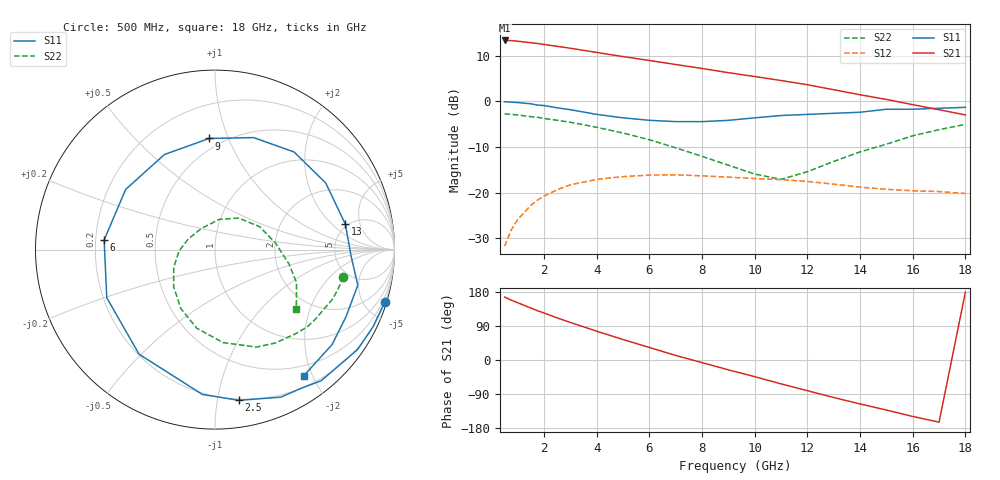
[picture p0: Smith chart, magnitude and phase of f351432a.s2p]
!ATF-35143
!S-PARAMETERS at Vds=2V  Id=5mA.  LAST UPDATED 06-3-99
# ghz s ma r 50
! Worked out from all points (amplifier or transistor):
!   23 points, 500 MHz to 18 GHz, reference 50 ohm
!   highest |S21| = 13.3 dB at 500 MHz (marker M1)
!   |S21| within 3 dB of that: start of sweep to 4.414 GHz
!   unconditionally stable (mu >= 1): 9.019 GHz to end of sweep
!   at 1.5 GHz: K = 0.17, MSG = 17.8 dB, |S12| = -22.7 dB
!   at 7 GHz: K = 0.78, MSG = 12.1 dB, |S12| = -16.1 dB
!   at 18 GHz: K = 1.55, MAG = 4.2 dB, |S12| = -20.2 dB
!   lowest NFmin = 0.10 dB at 500 MHz
!   S11 on the Smith chart (normalised r, x): 500 MHz: 0.23, -6.68; 2.5 GHz: 0.19, -1.15; 6 GHz: 0.23, +0.04; 9 GHz: 0.42, +0.85; 13 GHz: 4.77, +2.98; 18 GHz: 0.35, -1.87
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0.5  0.99 -17.0  4.64 166.0  0.026 78.0  0.73 -12.0
0.75  0.98 -26.0  4.62 158.0  0.039 71.0  0.72 -18.0
1  0.97 -35.0  4.55 151.0  0.051 66.0  0.71 -23.0
1.5  0.94 -51.0  4.38 137.0  0.073 55.0  0.68 -35.0
1.75  0.91 -58.0  4.3 130.0  0.083 50.0  0.67 -40.0
2.5  0.85 -81.0  4 111.0  0.108 35.0  0.62 -57.0
3  0.81 -95.0  3.81 99.0  0.122 25.0  0.59 -67.0
4  0.72 -126.0  3.43 76.0  0.14 7.0  0.52 -85.0
5  0.66 -156.0  3.09 54.0  0.15 -10.0  0.45 -103.0
6  0.62 175.0  2.8 33.0  0.156 -26.0  0.38 -120.0
7  0.6 146.0  2.53 12.0  0.157 -41.0  0.31 -138.0
8  0.6 118.0  2.29 -7.0  0.153 -54.0  0.25 -157.0
9  0.62 93.0  2.06 -26.0  0.148 -67.0  0.2 -178.0
10  0.66 71.0  1.87 -44.0  0.143 -78.0  0.16 158.0
11  0.7 51.0  1.69 -63.0  0.139 -89.0  0.14 122.0
12  0.72 31.0  1.52 -81.0  0.133 -100.0  0.17 82.0
13  0.74 11.0  1.34 -99.0  0.124 -111.0  0.22 53.0
14  0.76 -3.0  1.18 -116.0  0.115 -119.0  0.28 27.0
15  0.82 -14.0  1.05 -132.0  0.109 -127.0  0.34 6.0
16  0.82 -27.0  0.92 -149.0  0.105 -135.0  0.42 -11.0
17  0.84 -39.0  0.81 -164.0  0.103 -143.0  0.49 -22.0
18  0.86 -55.0  0.71 179.0  0.098 -152.0  0.56 -36.0
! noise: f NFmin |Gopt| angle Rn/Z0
0.5  0.1  0.91  6  0.22
0.9  0.12  0.87  15  0.22
1.5  0.2  0.81  28  0.22
1.8  0.23  0.78  33  0.21
2.5  0.33  0.71  50  0.19
3  0.39  0.66  62  0.17
5  0.64  0.52  114  0.09
6  0.77  0.47  143  0.06
8  1.02  0.41  -155  0.07
10  1.27  0.41  -90  0.24
